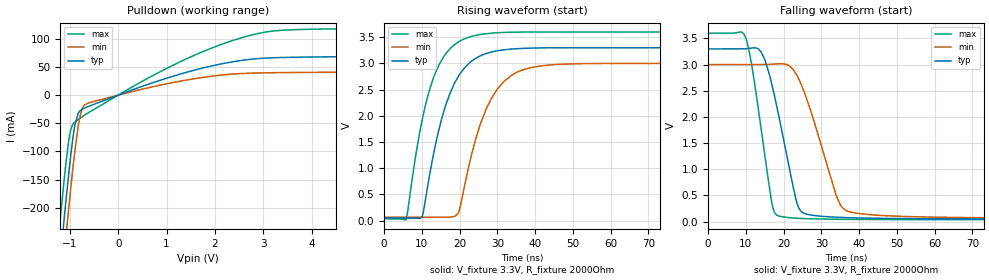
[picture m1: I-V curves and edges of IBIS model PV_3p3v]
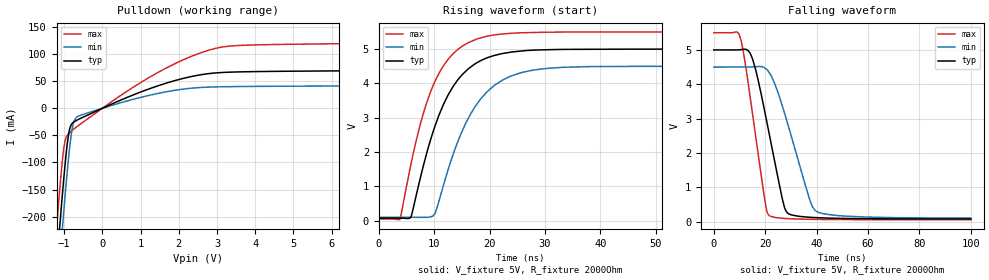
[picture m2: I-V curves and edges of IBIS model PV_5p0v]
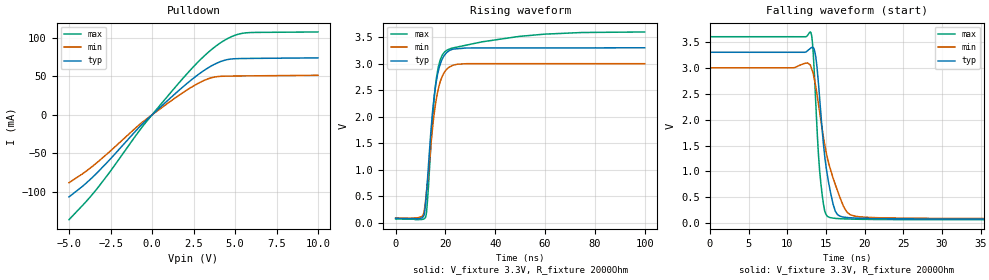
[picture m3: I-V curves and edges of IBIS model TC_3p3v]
|Texas Instruments Incorporated
|High or Low Side Measurement, Bi-directional Current adn Power
|Monitor with I2C Interface
| Marketing part#   Digital Voltage Range  Package   Pins
|INA3221   3.0 V to 5.5 V   QFN   16
[IBIS Ver]   4.0
[File name]   ina3221.ibs
[File Rev]   1.0
[Date]   05/09/2012
[Source]   Texas Instruments Incorporated.
   Analog-eLab, HPA
   12500 TI Blvd
   Dallas, TX -75243
   For Support e-mail: elab_ibis@list.ti.com
[Notes]   Revision History:
   1.0: 05/09/2012
   - Initial version of the model
   - Initial Model generated from simulations in TISPICED
   - Model names with a trailing _33 contains the model for
   3.3V (3V and 3.6V).
   _ Model names with trailing _5 contains
   the model for 5V (4.5V and 5.5V) operation.
   - Model not matched to measurements
   - C_comp although listed in numerical order of values are
   Obtained from varying PVT conditions. For PVT conditions
   for each specific value, refer the buffer description under
   respective [Model]. IBIS model user is responsible for using
   appropriate C_comp to simulate for Signal Integrity.
   - Combined Non-monotonic errors for SDA_33 and SDA_5 are minor
   and reflect SPICE transistor simulations
[Disclaimer]
  This model is designed as an aid for customers of Texas Instruments.
  TI and its licensors and suppliers make no warranties, either expressed
  or implied, with respect to this model, including the warranties of
  merchantability or fitness for a particular purpose.  The model is
  provided solely on an "as is" basis.  The entire risk as to its quality
  and performance is with the customer.
[Copyright] (C) Copyright 2012Texas Instruments Incorporated.
   All rights reserved.
|   INA3221
[Component]   ina3221
[Manufacturer] TI
[Package]   | 16 QFN package
| variable   typ   min   max
R_pkg  0.047   0.043   0.058
L_pkg  1.57nH  1.48nH  1.81nH
C_pkg  0.24pF  0.22pF  0.26pF
|-------------------------PIN------------------------------------------------
[Pin] signal_name  model_name  R_pin  L_pin C_pin
1   IN-3   TERM   NA   NA   NA
2   IN+3   TERM   NA   NA   NA
3   GND   GND   NA   NA   NA
4   VS   POWER   NA   NA   NA
5   A0   A0   NA   NA   NA
6   SCL   SCL   NA   NA   NA
7   SDA   SDA   NA   NA   NA
8   Warning ALERT   NA   NA   NA
9   CRITICAL ALERT   NA   NA   NA
10  PV   PV   NA   NA   NA
11  IN-1   TERM   NA   NA   NA
12  IN+1   TERM   NA   NA   NA
13  TC   TC   NA   NA   NA
14  IN-2   TERM   NA   NA   NA
15  IN-2   TERM   NA   NA   NA
16  VPU   TERM   NA   NA   NA
|   Model Selectors
[Model Selector]  PV
PV_3p3v  3V digital  open drain
PV_5p0v  5V digital  open drain
[Model Selector]  TC
TC_3p3v  3V digital  open drain
TC_5p0v  5V digital  open drain
[Model Selector]  A0
A0_33   3V digital input
A0_5   5V digital input
[Model Selector]  A1
A1_33   3V digital input
A1_5   5V digital input
[Model Selector]  SCL
SCL_33   3V digital input
SCL_5   5V digital input
[Model Selector]  ALERT
ALERT_33  3V digital open drain output
ALERT_5  5V digital open drain output
[Model Selector]  SDA
SDA_33  3V digital I/O open drain
SDA_5  5V digital I/O open drain
[Model Selector]  TERM
TERM_33  3V terminator
TERM_5  5V terminator
|   TERM Model
[Model] TERM_33
Model_type Terminator
C_comp   1e-20   1e-20   1e-20
| variable   typ   min   max
[Voltage Range]   3.3   3   3.6
|Ambient Temperature Range   27   85   -40
[Temperature Range]   30   88   -40
[Model] TERM_5
Model_type Terminator
C_comp   1e-20   1e-20   1e-20
| variable   typ   min   max
[Voltage Range]   5   4.5   5.5
|Ambient Temperature Range   27   85   -40
[Temperature Range]   30   88   -40
| Models and submodels in the file (16): PV_3p3v (Open_drain), PV_5p0v (Open_drain), TC_3p3v (Open_drain), TC_5p0v (Open_drain), A0_33 (Input), A0_5 (Input), A1_33 (Input), A1_5 (Input), SCL_33 (Input), SCL_5 (Input), ALERT_33 (Open_drain), ALERT_5 (Open_drain), SDA_33 (I/O_open_drain), SDA_5 (I/O_open_drain), TERM_33 (Terminator), TERM_5 (Terminator)
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|   PV_3p3v model
[Model]   PV_3p3v
Model_type   Open_drain
Polarity   Non-Inverting
Vmeas = 1.65
Vref = 3.3
Cref = 1pF
Rref = 2000
|   typ   min   max
C_comp   1.585pF   1.384pF   1.852pF
[Voltage Range]   3.3   3   3.6
[Temperature Range]   30   88   -40
[Pullup Reference]   3.3   3   3.6
[Pulldown Reference]   -0   -0   -0
[Power Clamp Reference]   3.3   3   3.6
[GND Clamp Reference]   -0   -0   -0
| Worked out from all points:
|   slope of the pulldown table from 0 to 0.495 V, typ, clamps not added: 31.9 ohm
|   falling waveform, V_fixture 3.3V, R_fixture 2000Ohm: 20-80 % time 5.64ns typ, 7.51ns min, 4.26ns max; typ from 3.3 V to 0.05 V
|   rising waveform, V_fixture 3.3V, R_fixture 2000Ohm: 20-80 % time 7.21ns typ, 7.83ns min, 6.64ns max; typ from 0.05 V to 3.3 V
[Pulldown]
|   Voltage   I(typ)   I(min)   I(max)
-3.3V     -2.337A    -2.398A    -2.27A
-1.211V   -304mA     -368.8mA   -231.9mA
-1.112V   -215.3mA   -279.1mA   -146.2mA
-1.082V   -189.6mA   -252.7mA   -122.5mA
-1.033V   -148.1mA   -209.6mA   -87.33mA
-993.3mV  -116.6mA   -176mA     -66.28mA
-894.3mV  -52.67mA   -98.28mA   -47.77mA
-755.7mV  -25.75mA   -26.73mA   -38.92mA
-547.8mV  -17.92mA   -12.38mA   -27.73mA
1.254V    36.6mA     24.35mA    58.11mA
2.779V    64mA       39.08mA    107.1mA
6.59V     69.43mA    41.42mA    119.7mA
[Ramp]
R_load = 2000
|   typ   min   max
dV/dt_r   1.95003/7.21191e-09   1.76025/7.83161e-09   2.13898/6.63657e-09
dV/dt_f   1.94998/5.64206e-09   1.75976/7.50776e-09   2.13898/4.26172e-09
[Falling Waveform]
V_fixture = 3.3V
V_fixture_min = 3V
V_fixture_max = 3.6V
R_fixture = 2000Ohm
C_fixture = 0F
|   Time   V(typ)   V(min)   V(max)
0s        3.3V       3V         3.6V
10.17ns   3.304V     3.001V     3.474V
14.19ns   3.228V     3.001V     1.712V
16.71ns   2.676V     3.006V     432.9mV
18.16ns   2.217V     3.013V     123.9mV
23.42ns   382.3mV    2.81V      63.32mV
24.51ns   202.6mV    2.649V     59.48mV
33.99ns   82.21mV    488.1mV    43.5mV
36.5ns    75.51mV    212.6mV    41.61mV
100ns     50.03mV    67.06mV    35.03mV
[Rising Waveform]
V_fixture = 3.3V
V_fixture_min = 3V
V_fixture_max = 3.6V
R_fixture = 2000Ohm
C_fixture = 0F
|   Time   V(typ)   V(min)   V(max)
0s        49.94mV    66.23mV    35.02mV
5.906ns   48.64mV    66.29mV    22.4mV
10.09ns   73.68mV    66.34mV    1.922V
15.13ns   1.915V     66.4mV     3.049V
18.73ns   2.635V     83.03mV    3.362V
20.27ns   2.818V     304mV      3.435V
23.48ns   3.062V     1.351V     3.523V
27.06ns   3.19V      2.136V     3.568V
35.02ns   3.281V     2.827V     3.598V
100ns     3.3V       3V         3.6V
|   PV_5p0v model
[Model]   PV_5p0v
Model_type   Open_drain
Polarity   Non-Inverting
Vmeas = 2.5
Vref = 5
Cref = 1pF
Rref = 2000
|   typ   min   max
C_comp   1.585pF   1.384pF   1.852pF
[Voltage Range]   5   4.5   5.5
[Temperature Range]   30   88   -40
[Pullup Reference]   5   4.5   5.5
[Pulldown Reference]   -0   -0   -0
[Power Clamp Reference]   5   4.5   5.5
[GND Clamp Reference]   -0   -0   -0
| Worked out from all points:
|   slope of the pulldown table from 0 to 0.75 V, typ, clamps not added: 32.6 ohm
|   falling waveform, V_fixture 5V, R_fixture 2000Ohm: 20-80 % time 7.99ns typ, 10.3ns min, 6.19ns max; typ from 5 V to 0.076 V
|   rising waveform, V_fixture 5V, R_fixture 2000Ohm: 20-80 % time 6.64ns typ, 7.2ns min, 6.11ns max; typ from 0.076 V to 5 V
[Pulldown]
|   Voltage   I(typ)   I(min)   I(max)
-5V       -4.023A    -4.081A    -3.958A
-1.25V    -339.7mA   -404.6mA   -267.1mA
-1.13V    -231.1mA   -295.1mA   -161mA
-1.04V    -153.9mA   -215.7mA   -91.9mA
-965mV    -95.67mA   -152.7mA   -56.97mA
-875mV    -44.48mA   -84.77mA   -46.38mA
-785mV    -27.53mA   -35.73mA   -40.66mA
-680mV    -22.51mA   -16.79mA   -34.63mA
1.06V     31.58mA    21.12mA    49.97mA
2.53V     61.38mA    38.25mA    101.3mA
8.26V     74.16mA    45.04mA    126.3mA
9.985V    89.62mA    55.88mA    149.7mA
[Ramp]
R_load = 2000
|   typ   min   max
dV/dt_r   2.95451/6.6415e-09   2.64021/7.2055e-09   3.26785/6.1071e-09
dV/dt_f   2.95441/7.99289e-09   2.63935/1.03196e-08   3.26785/6.19466e-09
[Falling Waveform]
V_fixture = 5V
V_fixture_min = 4.5V
V_fixture_max = 5.5V
R_fixture = 2000Ohm
C_fixture = 0F
|   Time   V(typ)   V(min)   V(max)
0s        5V         4.5V       5.5V
9.215ns   5.001V     4.501V     5.518V
10.45ns   5.008V     4.501V     5.32V
15.09ns   4.734V     4.506V     3.124V
19.53ns   3.312V     4.493V     770.2mV
21.71ns   2.496V     4.319V     166.5mV
28.12ns   300mV      3.008V     87.43mV
37.4ns    123.4mV    613.3mV    65.59mV
39.29ns   115.7mV    330.5mV    63.46mV
100ns     75.98mV    101.1mV    53.59mV
[Rising Waveform]
V_fixture = 5V
V_fixture_min = 4.5V
V_fixture_max = 5.5V
R_fixture = 2000Ohm
C_fixture = 0F
|   Time   V(typ)   V(min)   V(max)
0s        75.81mV    99.63mV    53.57mV
3.827ns   73.28mV    98.78mV    38.66mV
5.873ns   130.2mV    98.32mV    1.69V
7.977ns   1.549V     97.85mV    3.085V
9.829ns   2.601V     137.9mV    3.942V
13.38ns   3.901V     1.907V     4.859V
17.91ns   4.62V      3.441V     5.307V
22.34ns   4.872V     4.099V     5.441V
30.84ns   4.984V     4.445V     5.494V
100ns     5V         4.5V       5.5V
|   TC_3p3v model
[Model]   TC_3p3v
Model_type   Open_drain
Polarity   Non-Inverting
Vmeas = 1.65
Vref = 3.3
Cref = 1pF
Rref = 2000
|   typ   min   max
C_comp   0.609pF   0.575pF   0.639pF
[Voltage Range]   3.3   3   3.6
[Temperature Range]   30   88   -40
[Pullup Reference]   3.3   3   3.6
[Pulldown Reference]   -0   -0   -0
[Power Clamp Reference]   3.3   3   3.6
[GND Clamp Reference]   -0   -0   -0
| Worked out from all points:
|   slope of the pulldown table from 0 to 0.495 V, typ, clamps not added: 50.2 ohm
|   falling waveform, V_fixture 3.3V, R_fixture 2000Ohm: 20-80 % time 1.37ns typ, 2.47ns min, 837ps max; typ from 3.3 V to 0.08 V
|   rising waveform, V_fixture 3.3V, R_fixture 2000Ohm: 20-80 % time 3.65ns typ, 4.08ns min, 3.67ns max; typ from 0.08 V to 3.3 V
[Pulldown]
|   Voltage   I(typ)   I(min)   I(max)
-5V       -106.4mA   -87.9mA    -135.8mA
-4.16V    -92.07mA   -76mA      -116.8mA
-3.26V    -74.05mA   -60.91mA   -94.26mA
-2.465V   -56.14mA   -45.98mA   -71.79mA
-635mV    -12.93mA   -10.42mA   -16.83mA
835mV     16.57mA    13.3mA     21.52mA
2.545V    48.33mA    38.03mA    63.49mA
3.16V     57.93mA    44.82mA    76.65mA
3.775V    65.68mA    49.02mA    87.92mA
4.615V    71.86mA    50.17mA    99.51mA
5.47V     72.93mA    50.38mA    105.7mA
9.985V    73.75mA    51.21mA    107.3mA
[Ramp]
R_load = 2000
|   typ   min   max
dV/dt_r   1.93162/3.64368e-09   1.74584/4.07898e-09   2.11832/3.67241e-09
dV/dt_f   1.93175/1.36703e-09   1.74588/2.47474e-09   2.11911/8.37074e-10
[Falling Waveform]
V_fixture = 3.3V
V_fixture_min = 3V
V_fixture_max = 3.6V
R_fixture = 2000Ohm
C_fixture = 0F
|   Time   V(typ)   V(min)   V(max)
0s        3.3V       3V         3.6V
13.07ns   3.383V     3.02V      3.678V
13.38ns   3.388V     2.878V     3.243V
13.71ns   3.199V     2.628V     2.284V
14.35ns   2.123V     1.986V     771.6mV
14.84ns   1.309V     1.526V     244.2mV
15.62ns   586mV      1.029V     106.6mV
17.71ns   111mV      217.1mV    82.21mV
19.85ns   94.13mV    118.6mV    75.07mV
100ns     80.4mV     90.17mV    68.13mV
[Rising Waveform]
V_fixture = 3.3V
V_fixture_min = 3V
V_fixture_max = 3.6V
R_fixture = 2000Ohm
C_fixture = 0F
|   Time   V(typ)   V(min)   V(max)
0s        80.39mV    90.17mV    68.12mV
10.39ns   86.38mV    111.8mV    59.41mV
11.53ns   165.8mV    237.7mV    74.58mV
12.1ns    411.5mV    448.5mV    113.2mV
12.99ns   943.3mV    856mV      547.7mV
14.67ns   2.008V     1.711V     1.85V
16.5ns    2.712V     2.372V     2.766V
18.76ns   3.09V      2.766V     3.165V
21.7ns    3.251V     2.94V      3.278V
100ns     3.3V       3V         3.599V
